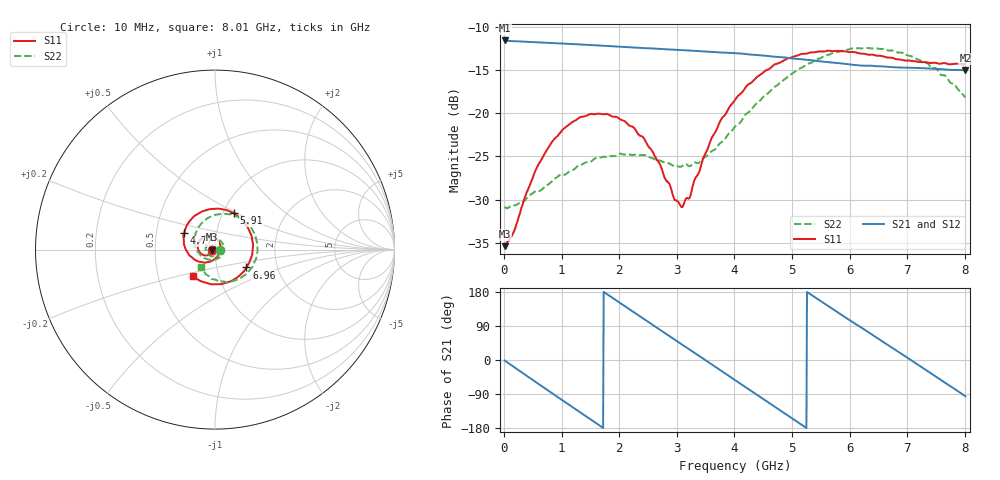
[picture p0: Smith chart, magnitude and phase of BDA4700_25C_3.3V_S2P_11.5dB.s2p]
!Agilent Technologies,E5071B,MY42404982,A.09.10
!Date: Mon Oct 20 18:07:51 2025
!Data & Calibration Information:
!Freq	S11:SOLT2(ON)	S21:SOLT2(ON)	S12:SOLT2(ON)	S22:SOLT2(ON)
# Hz S RI R 50
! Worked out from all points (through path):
!   801 points, 10 MHz to 8.01 GHz, reference 50 ohm
!   highest |S21| = -11.61 dB at 10 MHz (marker M1); lowest = -15.0 dB at 8.01 GHz (marker M2)
!   group delay of S21, straight-line fit = 282 ps
!   lowest |S11| = -35.4 dB at 10 MHz (marker M3), VSWR 1.03, Z = 48.3 - j0.101 ohm
!   |S11| at or under -10 dB: start of sweep to end of sweep
!   |S22| runs from -31.0 to -12.5 dB; largest |S21 - S12| = 0.003
!   S11 on the Smith chart (normalised r, x): 10 MHz: 0.97, -0.00; 4.77 GHz: 0.70, +0.13; 5.91 GHz: 1.13, +0.48; 6.96 GHz: 1.39, -0.29; 8.01 GHz: 0.75, -0.23
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1e7  -0.017 -0.00105  0.2627 -0.00573  0.2626 -0.00598  0.0287 -0.00145
1.6e8  -0.0179 -0.00969  0.2487 -0.077  0.2487 -0.077  0.0277 -0.00942
5.3e8  -0.0347 -0.0291  0.144 -0.2128  0.1437 -0.2129  0.0137 -0.0325
7.2e8  -0.0495 -0.0329  0.0627 -0.2472  0.0628 -0.2471  -0.00168 -0.0378
1.35e9  -0.0952 0.00555  -0.1934 -0.1565  -0.1935 -0.1567  -0.05 -0.00659
1.93e9  -0.068 0.0669  -0.2269 0.0862  -0.2269 0.0861  -0.0267 0.0498
2.26e9  -0.029 0.0768  -0.1385 0.195  -0.1387 0.195  0.0105 0.0565
2.68e9  0.0186 0.0489  0.0303 0.2332  0.0299 0.2331  0.0471 0.0249
2.96e9  0.0295 0.0114  0.136 0.1881  0.1358 0.1878  0.0489 -0.00811
3.1e9  0.0273 -0.00897  0.1779 0.1474  0.1768 0.1484  0.0427 -0.0255
3.23e9  0.0202 -0.0261  0.2053 0.1032  0.2054 0.1028  0.0323 -0.0375
3.54e9  -0.015 -0.061  0.2259 -0.0194  0.2259 -0.0197  -0.00565 -0.0572
4.01e9  -0.102 -0.0616  0.1339 -0.177  0.134 -0.1766  -0.0749 -0.0365
4.39e9  -0.1615 -0.00256  -0.00658 -0.2164  -0.00647 -0.217  -0.1114 0.0247
4.77e9  -0.1714 0.0913  -0.1375 -0.16  -0.1365 -0.1608  -0.1005 0.1079
5.35e9  -0.0669 0.214  -0.1988 0.0336  -0.199 0.0325  0.0191 0.1956
5.91e9  0.105 0.2022  -0.0786 0.1762  -0.0793 0.1756  0.1763 0.148
6.3e9  0.1888 0.11  0.0451 0.1825  0.0468 0.1811  0.234 0.0403
6.68e9  0.2087 -0.0143  0.1457 0.1138  0.1462 0.1135  0.2178 -0.075
6.96e9  0.1752 -0.0995  0.1803 0.0329  0.1802 0.0319  0.1691 -0.1406
7.48e9  0.0361 -0.1922  0.1338 -0.1207  0.1338 -0.1211  0.0251 -0.1804
8.01e9  -0.1238 -0.1472  -0.0177 -0.176  -0.0171 -0.1762  -0.0782 -0.0949
